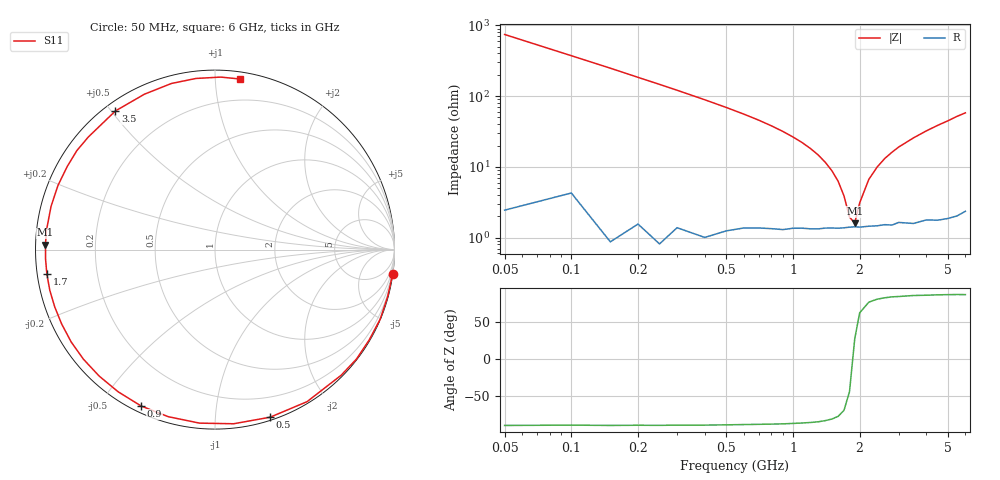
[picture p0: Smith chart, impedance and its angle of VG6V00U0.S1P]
! Infineon Technologies  Discrete & RF Semiconductors
! BB 831
! Si Tuning Diode in SOD323
! VR = 6 V
! S-Parameters:  July  1999
# GHz  S  MA  R  50
!  f  S11
! GHz  MAG  ANG
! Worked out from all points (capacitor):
!   34 points, 50 MHz to 6 GHz, reference 50 ohm
!   read as one part to ground: C = 4.26 pF near 50 MHz
!   lowest |Z| = 1.6 ohm at 1.9 GHz (marker M1)
!   series resonance near 1.865 GHz, so ESL is about 1.7 nH
!   S11 on the Smith chart (normalised r, x): 50 MHz: 0, -15; 500 MHz: 0.02, -1.38; 900 MHz: 0.03, -0.63; 1.7 GHz: 0.03, -0.07; 3.5 GHz: 0.03, +0.51; 6 GHz: 0.05, +1.16
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0.05  0.9996 -7.7
0.15  0.9986 -22.8
0.25  0.9966 -37.7
0.3  0.992 -44.9
0.4  0.9904 -58.8
0.5  0.983 -71.8
0.6  0.9759 -83.9
0.7  0.9707 -95.1
0.8  0.9666 -105.6
0.9  0.9637 -115.3
1  0.9585 -124.3
1.1  0.9555 -132.5
1.2  0.954 -140.2
1.3  0.9523 -147.3
1.4  0.9496 -154.1
1.6  0.9479 -166.1
1.7  0.9467 -171.7
1.9  0.9448 178.3
2.2  0.9447 165.2
2.4  0.9451 157.7
2.6  0.9446 150.6
3  0.9444 138.4
3.5  0.9511 125.7
4  0.951 114.4
4.5  0.9568 104.7
5  0.9594 96.4
5.5  0.9616 88.1
6  0.9606 81.6
